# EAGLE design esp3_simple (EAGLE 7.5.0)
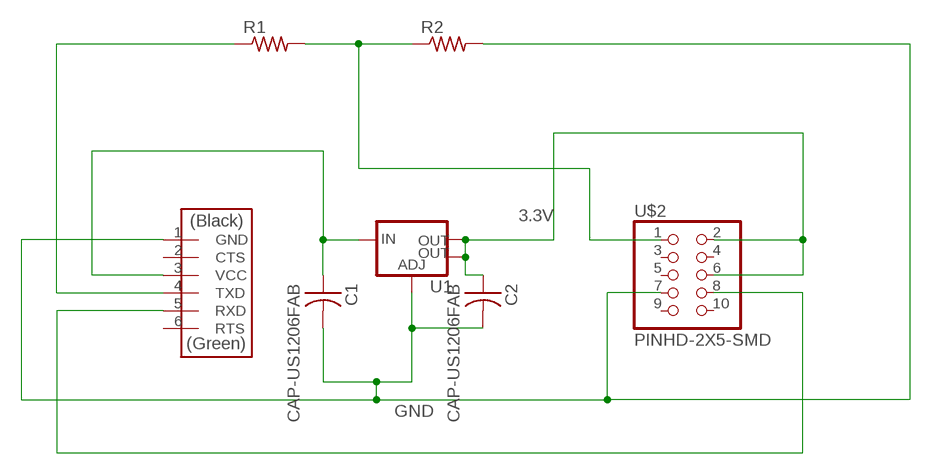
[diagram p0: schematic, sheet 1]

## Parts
C1  CAP-US1206FAB  [C1206FAB]
C2  CAP-US1206FAB  [C1206FAB]
R1  RES-US1206FAB  [R1206FAB]
R2  RES-US1206FAB  [R1206FAB]
U1  V_REG_LM1117SOT223  [SOT223]
U$1  FTDI-SMD-HEADER  [1X06SMD]
U$2  PINHD-2X5-SMD  [2X05SMD]

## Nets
3.3V: C2.1 U1.2(OUT) U1.4(OUT) U$2.2 U$2.6
GND: C1.2 C2.2 R2.2 U1.1(ADJ) U$1.1(GND) U$2.7
N$1: R1.2 R2.1 U$2.1
N$2: C1.1 U1.3(IN) U$1.3(VCC)
N$3: R1.1 U$1.4(TXD)
N$4: U$1.5(RXD) U$2.8
Unconnected: U$1.2(CTS) U$1.6(RTS) U$2.3 U$2.4 U$2.5 U$2.9 U$2.10

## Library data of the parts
C1 C2 = fab:CAP-US
R1 R2 = fab:RES-US: Resistor (US Symbol)
U1 = fab:V_REG_LM1117: Voltage Regulator LM1117 Standard adjustable voltage regulator but in SMD form. Spark Fun Electronics SKU : COM-00595; PROD_ID: VREG-08170
U$1 = fab:FTDI-SMD-HEADER
U$2 = fab:PINHD-2X5-SMD

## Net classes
0 default: width 0.33 mm, drill 0.254 mm, clearance 0.406 mm

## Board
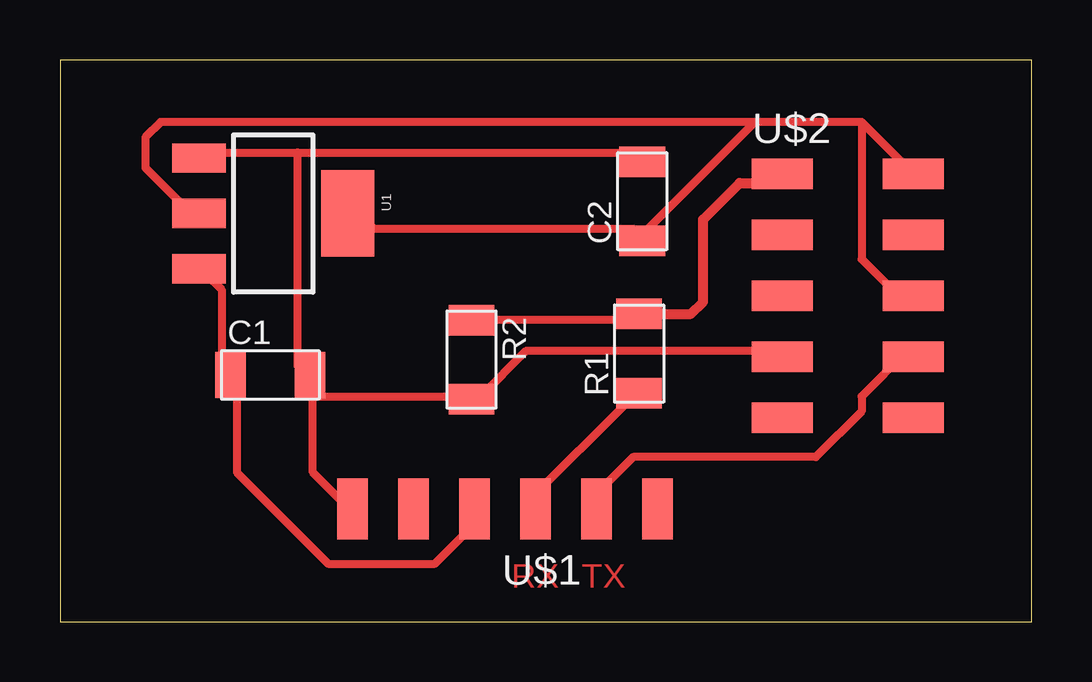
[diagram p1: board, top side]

Size 40.49 x 23.42 mm. Coordinates in mm from the lower left corner, seen from the top.
Outline: 0,0 40.49,0 40.49,23.42 0,23.42 0,0
Copper layers (1*16): Top 0.035mm / dielectric 1.5mm / Bottom 0.035mm
Design rules "default *": minimum track width 10mil, minimum drill 24mil, track to track 16mil, track to pad 16mil, pad to pad 16mil, via to via 16mil, smd to smd 16mil, copper to edge 40mil, drill to drill 8mil, minimum pad ring 10mil, minimum via ring 8mil, stop-mask expansion 4mil, vias tented up to drill 0mil, thermal gap 10mil

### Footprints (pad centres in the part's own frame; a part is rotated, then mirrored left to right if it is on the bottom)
C1206FAB = smd 1.27 x 1.905: 1 -1.651,0; 2 1.651,0
R1206FAB = smd 1.27 x 1.905: 1 -1.651,0; 2 1.651,0
SOT223 = smd 1.219 x 2.235: 1 -2.311,-3.099; 2 0,-3.099; 3 2.311,-3.099 | smd 3.6 x 2.2: 4 0,3.099
1X06SMD = smd 2.54 x 1.27: 1 0,6.35; 2 0,3.81; 3 0,1.27; 4 0,-1.27; 5 0,-3.81; 6 0,-6.35
2X05SMD = smd 2.54 x 1.27: 1 -2.54,2.54; 2 2.92,2.54; 3 -2.54,0; 4 2.92,0; 5 -2.54,-2.54; 6 2.92,-2.54; 7 -2.54,-5.08; 8 2.92,-5.08; 9 -2.54,-7.62; 10 2.92,-7.62

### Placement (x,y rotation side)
C1  8.76,10.29 0 top
C2  24.26,17.53 90 top
R1  24.13,11.18 90 top
R2  17.14,10.92 270 top
U1  8.89,17.02 270 top
U$1  18.54,4.7 90 top
U$2  32.64,16.13 0 top

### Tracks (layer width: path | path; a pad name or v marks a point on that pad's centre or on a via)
3.3V
  Top 0.33: U1.4 12.45,17.02 13.08,16.38 23.88,16.38 C2.1 24.51,16.38 28.96,20.83 | 33.4,20.83 28.96,20.83 | 28.96,20.83 4.19,20.83 3.56,20.19 3.56,18.92 5.46,17.02 U1.2 | 33.4,20.83 35.31,18.92 U$2.2 | 33.4,20.83 33.4,15.11 34.67,13.84 35.31,13.84 U$2.6
GND
  Top 0.33: 9.91,19.56 6.1,19.56 U1.1 | 9.91,19.56 23.88,19.56 C2.2 | 10.54,9.4 10.54,6.22 11.81,4.95 U$1.1 | 10.54,9.4 10.54,10.03 C1.2 | 10.54,9.4 16.89,9.4 R2.2 17.53,9.4 19.43,11.3 29.59,11.3 U$2.7 | 10.54,9.4 C1.2 | 9.91,19.56 9.91,10.67 C1.2
N$1
  Top 0.33: R2.1 23.88,12.57 R1.2 | 28.96,18.29 29.59,18.29 U$2.1
  Top 0.406: R1.2 26.29,12.83 26.8,13.34 26.8,16.76 28.32,18.29 29.72,18.29 U$2.1
N$2
  Top 0.33: U1.3 6.1,14.48 6.73,13.84 6.73,10.67 C1.1 7.37,10.03 7.37,6.22 11.18,2.41 15.62,2.41 16.89,3.68 16.89,4.32 U$1.3
N$3
  Top 0.33: R1.1 23.88,9.4 19.43,4.95 U$1.4
N$4
  Top 0.33: U$1.5 22.61,4.95 22.61,5.59 23.88,6.86 31.5,6.86 33.4,8.76 33.4,9.4 35.31,11.3 U$2.8

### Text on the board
Top: RX | TX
